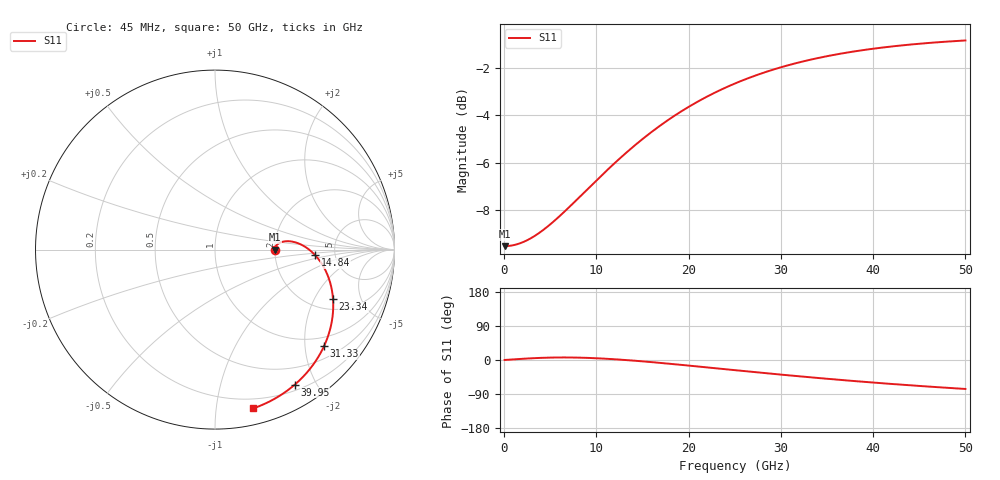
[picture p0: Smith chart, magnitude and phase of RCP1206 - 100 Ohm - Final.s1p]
!Vishay Electro-Films Inc.
!RCP Family
!Case Size 1206
!Assembly Style Surface Mount
!11/2/2015
!efi@vishay.com
# GHz S MA R 50
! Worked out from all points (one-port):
!   801 points, 45 MHz to 50 GHz, reference 50 ohm
!   lowest |S11| = -9.5 dB at 45 MHz (marker M1), VSWR 2.00, Z = 100 + j0.1 ohm
!   |S11| at or under -10 dB: nowhere
!   S11 on the Smith chart (normalised r, x): 45 MHz: 2.00, +0.00; 14.84 GHz: 3.51, -0.32; 23.34 GHz: 2.54, -2.85; 31.33 GHz: 0.77, -2.42; 39.95 GHz: 0.27, -1.72; 50 GHz: 0.12, -1.26
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0.045  0.3333 0.1
1.418762  0.3366 2.4
2.854969  0.3462 4.4
4.54095  0.3647 6.1
6.289375  0.3905 6.7
7.912913  0.419 6.4
9.474006  0.449 5.2
11.0351  0.4806 3.3
12.53375  0.5116 1.0
13.65774  0.5349 -0.9
14.84417  0.5593 -3.2
16.71748  0.5968 -7.2
18.77812  0.636 -11.9
21.08854  0.6769 -17.3
23.33652  0.713 -22.8
25.0225  0.7377 -26.8
26.52115  0.7578 -30.4
28.0198  0.7763 -34.0
29.58089  0.7939 -37.6
31.26687  0.811 -41.4
31.32932  0.8116 -41.6
34.45151  0.8386 -48.4
37.51125  0.8599 -54.7
39.94656  0.8738 -59.4
41.81987  0.8829 -62.9
43.75563  0.891 -66.3
46.87781  0.9017 -71.6
50  0.91 -76.4
